FUNCTION_BLOCK PQDXXA_PARA
TITLE =PN Driver
AUTHOR : Parker
VERSION : 0.2


VAR_INPUT
  INIT : BOOL ;	//initilaize after Start / Baustein initialisieren
  READ_ALL : BOOL ;	//read out all parameters / alle Parameter auslesen
  WRITE_ALL : BOOL ;	//write all parameters / alle Parameter schreiben
  WRITE_SEL : BOOL ;	//write only selection parameters / nur die Auswahlparameter schreiben
  SINGLE_READ : BOOL ;	//read single parameter / einzelnen Wert lesen
  SINGLE_WRITE : BOOL ;	//write single parameter / einezelnen Wert schreiben
  SINGLE_INDEX : WORD ;	//parameter address / Adresse
  SAVE : BOOL ;	//save parameters in the module / Parameter im Modul speichern
  DEFAULT : BOOL ;	//set all parameters to the default setting / alle Parameter auf Werkseinstellung
  LOADBACK : BOOL ;	//load back the last saved parameter set / letzten gespeicheten Parametersatz zur
  PAR_CHANGE_OUT : STRUCT
   PARA_READY : BOOL ;
   BUS_VALID : BOOL ;
   ENABLE : BOOL ;	//Enable Signal for the Controller
   PARA_ACTIVE : BOOL ;
   PARVAL : DWORD ;	//Read out Value
  END_STRUCT ;
END_VAR
VAR_OUTPUT
  STATUS : INT ;	//0 = no active, 1 = ready and intitialized, 2 = busy, 3 = error / 0 = inaktiv, 1
  ERROR_LINE : INT ;	//number of the faulty parameter (range test or timeout) / Nummer des fehlerhafte
  DISC_LINE : INT ;	//line of 1st deviation / Zeile mit der ersten Abweichung
  DISC_COUNT : INT ;	//number of deriving parameters / Zahl der abweichenden Parameter
  PAR_CHANGE_IN : STRUCT
   PARVAL : DWORD ;
   PARAMODE : BOOL ;
   ADDRESS : WORD ;
   PARAVALID : BOOL ;
   PARAREAD : BOOL ;
   READULIM : BOOL ;
   READLLIM : BOOL ;
  END_STRUCT ;
END_VAR
VAR_IN_OUT
  PVSEL : INT ;	//Pump displacement selection [cm³/rev] / Auswahl des Verdrängungsvolumen [cm³/re
  PTYPE : INT ;	//1=F (swivel angle ctrl.), 2=P (+ open loop pressure ctrl.), 3=Q (+ closed loop
  CO : INT ;	//Selection of control option: 1=FP*/UP*, 2=FD*/UD* / Auswahl der Regleroption: 1
  DSP_VALVE : INT ;	//Pressure valve design series 2 = "11", 1 = "12"/ Konstruktionsstand des Druckve
  PSENSOR : INT ;	//Sensor nominal pressure in bar / Sensor Nenndruck in bar
  PNOMINAL : INT ;	//System pressure value in bar / Systemdruck in bar
  PCORR : INT ;	//Differential pressure setting in bar / Differenzdruckeinstellung in bar
  PLRPM : INT ;	//Engine speed in rpm / Motordrehzahl in U/min
  PLPL : INT ;	//Power limitation in 0,1kW / Leistungsgrenze in 0,1kW
  QCORR : INT ;	//Automatic flow correction in 0,01% / Automatische Volumenstromkorrektur in 0,01
  AQUP : DINT ;	//Ramp time up stroking (flow) for 0... 100% in ms / Rampenzeit aufschwenken (Vol
  AQDOWN : DINT ;	//Ramp time down stroking (flow) for 0... 100% in ms / Rampenzeit abschwenken (Vo
  APUP : DINT ;	//Ramp time (pressure up) for 0... 100% in ms / Rampenzeit (Druckanstieg) für 0..
  APDOWN : DINT ;	//Ramp time (pressure down) for 0... 100% in ms / Rampenzeit (Druckreduzierung) f
  MINXQ : INT ;	//Input scaling of the swivel angle sensor signal in mV / Eingangsskalierung des
  MAXXQ : INT ;	//Input scaling of the swivel angle sensor signal in mV / Eingangsskalierung des
  AINXQ : INT ;	//Input signal switching, swivel angel sensor, voltage (1) or current (2)/ Eingan
  AINXP : INT ;	//Input signal switching pressure sensor, voltage (1) or current (2) / Eingangssi
  CQFF : INT ;	//Offset swivel angle controller in 0,01% / Offset des Schwenkwinkelreglers in 0,
  CQP : INT ;	//P gain in 0,01 units / P-Anteil, Verstärkung in 0,01 Einheiten
  CQI : INT ;	//I gain in 0,1ms / I-Anteil, Nachstellzeit in 0,1ms
  CQILIM : INT ;	//I gain limitation in 0,01% / I-Anteil, Begegrenzung in 0,01%
  CQIC : INT ;	//I gain activation in 0,01% / I-Anteil, Aktivierung in 0,01%
  CQD : INT ;	//D gain in 0,1ms / D-Anteil, Vorhaltezeit in 0,1ms
  CQT1 : INT ;	//D gain filter in 0,1ms / D-Anteil, Filter in 0,1ms
  CPFF : INT ;	//Feed forward pressure valve in 0,01% / Vorsteuerwert des Druckventils in 0,01%
  CPP : INT ;	//P gain in 0,01 units / P-Anteil, Verstärkung in 0,01 Einheiten
  CPI : INT ;	//I gain in 0,1ms / I-Anteil, Nachstellzeit in 0,1ms
  CPILIM : INT ;	//I gain limitation in 0,01% / I-Anteil, Begrenzung in 0,01%
  CPIC : INT ;	//I gain activation in 0,01% / I-Anteil, Aktivierung in 0,01%
  CPD : INT ;	//D gain in 0,1ms / D-Anteil, Vorhaltezeit in 0,1ms
  CPT1 : INT ;	//D gain filter in 0,1ms / D-Anteil, Filter in 0,1ms
  CQMINVA : INT ;	//Compensation of the swivel angle valve deadband in mA / Kompensation der positi
  CQMINVB : INT ;	//Compensation of the swivel angle valve deadband in mA / Kompensation der positi
  CQMAXVA : INT ;	//Nominal current of the swivel angle valve in mA / Nennstrom des Schwenkwinkelve
  CQMAXVB : INT ;	//Nominal current of the swivel angle valve in mA / Nennstrom des Schwenkwinkelve
  TRIGGERQ : INT ;	//Trigger point of the swivel angel valve MIN function in 0,01% / Triggerpunkt de
  OFFSETQ : INT ;	//Offset function for neutral point adjustment of the directional valve in 0,01%
  CPMINV : INT ;	//Response threshold of the pressure valve in mA / Ansprechschwelle des Druckvent
  CPMAXV : INT ;	//Nominal current of the pressure valve in mA / Nennstrom des Druckventils in mA
  TRIGGERP : INT ;	//Trigger point of the pressure valve MIN function in 0,01% / Triggerpunkt der MI
  DFREQQ : INT ;	//Dither frequency in Hz / Dither Frequenz in Hz
  DAMPLQ : INT ;	//Dither amplitude in 0,01% of the rated current / Dither Amplitude in 0,01% des
  PWMQ : INT ;	//PWM Frequenz in Hz: 1-17 = 100|120|150|200|269|372|488|624|781|976|1201|1420|15
  PPWMQ : INT ;	//P gain of the current controller / P Verstärkung des Stromreglers
  IPWMQ : INT ;	//I gain of the current controller / I Verstärkung des Stromreglers
  DFREQP : INT ;	//Dither frequency in Hz / Dither Frequenz in Hz
  DAMPLP : INT ;	//Dither amplitude in 0,01% of the rated current / Dither Amplitude in 0,01% des
  PWMP : INT ;	//PWM Frequenz in Hz: 1-17 = 100|120|150|200|269|372|488|624|781|976|1201|1420|15
  PPWMP : INT ;	//P gain of the current controller / P Verstärkung des Stromreglers
  IPWMP : INT ;	//I gain of the current controller / I Verstärkung des Stromreglers
  SINGLEACCESS : DINT ;
END_VAR
VAR
  PARAINFO : ARRAY  [1 .. 51 ] OF STRUCT
   MINV : INT ;
   MAXV : INT ;
   VALUE : INT ;
   ADDRESS : WORD  := W#16#2001;
  END_STRUCT ;
  PARAINFO_LONG : ARRAY  [1 .. 4 ] OF STRUCT
   MINV : DINT ;
   MAXV : DINT ;
   VALUE : DINT ;
  END_STRUCT ;
  INTERNAL_STATE : INT ;
  SUBSTATE : INT ;
  i : INT ;
  actWaitCycles : INT ;
  oldParaReadVal : DWORD ;
  oldREADALL : BOOL ;
  oldWRITESEL : BOOL ;
  oldWRITEALL : BOOL ;
  oldPARAREADY : BOOL ;
  oldSINGLEWRITE : BOOL ;
  oldSINGLEREAD : BOOL ;
  oldSAVE : BOOL ;
  oldDEFAULT : BOOL ;
  oldLOADBACK : BOOL ;
  defaultFlag : BOOL ;
  saveFlag : BOOL ;
  readInEAFlag : BOOL ;
  readOnlyValues : BOOL ;
  initReceived : BOOL ;
  writeLimit : INT ;
  copyValue : INT ;
  copyValueLong : DINT ;
  discCountTemp : INT ;
  Displacement : ARRAY  [1 .. 15 ] OF
  INT  := 16, 20, 23, 28, 32, 40, 46, 63, 80, 92, 140, 180, 270, 360, 0;
END_VAR
VAR_TEMP
  MemFkt : INT ;
  PCI_DEFAULT : STRUCT
   PARVAL : DWORD ;
   PARAMODE : BOOL ;
   ADDRESS : WORD ;
   PARAVALID : BOOL ;
   PARAREAD : BOOL ;
   READULIM : BOOL ;
   READLLIM : BOOL ;
  END_STRUCT ;
  k : INT ;
  tmpDiff : DINT ;
  repeatFlag : BOOL ;
  tmpBool : BOOL ;
END_VAR
BEGIN
NETWORK
TITLE =SCL network
      SET   ;
      SAVE  ;
      =     L     18.3;
A7d0: CLR   ;
      =     #repeatFlag;
      U     #PAR_CHANGE_OUT.BUS_VALID;
      NOT   ;
      SPBN  A7d1;
      L     5;
      T     #INTERNAL_STATE;
      L     0;
      T     #SUBSTATE;
A7d1: L     #INTERNAL_STATE;
      L     20;
      <>I   ;
      SPBN  A7d2;
      L     0;
      T     #DISC_COUNT;
      L     -1;
      T     #DISC_LINE;
A7d2: CLR   ;
      U     #initReceived;
      NOT   ;
      U     #INIT;
      SPBN  A7d3;
      L     0;
      T     #INTERNAL_STATE;
      SET   ;
      =     #initReceived;
A7d3: L     #INTERNAL_STATE;
      L     0;
      TAK   ;
      ==I   ;
      T     LW    20;
      SPB   A7d5;
      SPA   A7d6;
A7d5: L     W#16#2001;
      T     #PARAINFO[1].ADDRESS;
      L     W#16#2002;
      T     #PARAINFO[2].ADDRESS;
      L     W#16#2003;
      T     #PARAINFO[3].ADDRESS;
      L     W#16#2004;
      T     #PARAINFO[4].ADDRESS;
      L     W#16#2011;
      T     #PARAINFO[5].ADDRESS;
      L     W#16#2012;
      T     #PARAINFO[6].ADDRESS;
      L     W#16#2013;
      T     #PARAINFO[7].ADDRESS;
      L     W#16#2014;
      T     #PARAINFO[8].ADDRESS;
      L     W#16#2015;
      T     #PARAINFO[9].ADDRESS;
      L     W#16#2016;
      T     #PARAINFO[10].ADDRESS;
      L     W#16#2021;
      T     #PARAINFO[11].ADDRESS;
      L     W#16#2022;
      T     #PARAINFO[12].ADDRESS;
      L     W#16#2023;
      T     #PARAINFO[13].ADDRESS;
      L     W#16#2024;
      T     #PARAINFO[14].ADDRESS;
      L     W#16#2025;
      T     #PARAINFO[15].ADDRESS;
      L     W#16#2026;
      T     #PARAINFO[16].ADDRESS;
      L     W#16#2027;
      T     #PARAINFO[17].ADDRESS;
      L     W#16#2028;
      T     #PARAINFO[18].ADDRESS;
      L     W#16#2031;
      T     #PARAINFO[19].ADDRESS;
      L     W#16#2032;
      T     #PARAINFO[20].ADDRESS;
      L     W#16#2033;
      T     #PARAINFO[21].ADDRESS;
      L     W#16#2034;
      T     #PARAINFO[22].ADDRESS;
      L     W#16#2039;
      T     #PARAINFO[23].ADDRESS;
      L     W#16#2036;
      T     #PARAINFO[24].ADDRESS;
      L     W#16#2037;
      T     #PARAINFO[25].ADDRESS;
      L     W#16#2041;
      T     #PARAINFO[26].ADDRESS;
      L     W#16#2042;
      T     #PARAINFO[27].ADDRESS;
      L     W#16#2043;
      T     #PARAINFO[28].ADDRESS;
      L     W#16#2044;
      T     #PARAINFO[29].ADDRESS;
      L     W#16#2045;
      T     #PARAINFO[30].ADDRESS;
      L     W#16#2046;
      T     #PARAINFO[31].ADDRESS;
      L     W#16#2047;
      T     #PARAINFO[32].ADDRESS;
      L     W#16#2051;
      T     #PARAINFO[33].ADDRESS;
      L     W#16#2052;
      T     #PARAINFO[34].ADDRESS;
      L     W#16#2053;
      T     #PARAINFO[35].ADDRESS;
      L     W#16#2054;
      T     #PARAINFO[36].ADDRESS;
      L     W#16#2055;
      T     #PARAINFO[37].ADDRESS;
      L     W#16#2056;
      T     #PARAINFO[38].ADDRESS;
      L     W#16#2061;
      T     #PARAINFO[39].ADDRESS;
      L     W#16#2062;
      T     #PARAINFO[40].ADDRESS;
      L     W#16#2063;
      T     #PARAINFO[41].ADDRESS;
      L     W#16#2071;
      T     #PARAINFO[42].ADDRESS;
      L     W#16#2072;
      T     #PARAINFO[43].ADDRESS;
      L     W#16#2073;
      T     #PARAINFO[44].ADDRESS;
      L     W#16#2074;
      T     #PARAINFO[45].ADDRESS;
      L     W#16#2075;
      T     #PARAINFO[46].ADDRESS;
      L     W#16#2081;
      T     #PARAINFO[47].ADDRESS;
      L     W#16#2082;
      T     #PARAINFO[48].ADDRESS;
      L     W#16#2083;
      T     #PARAINFO[49].ADDRESS;
      L     W#16#2084;
      T     #PARAINFO[50].ADDRESS;
      L     W#16#2085;
      T     #PARAINFO[51].ADDRESS;
      CLR   ;
      =     #saveFlag;
      L     5;
      T     #INTERNAL_STATE;
      SPA   A7d4;
A7d6: L     5;
      L     LW    20;
      ==I   ;
      SPB   A7d7;
      SPA   A7d8;
A7d7: CLR   ;
      U     #PAR_CHANGE_OUT.BUS_VALID;
      SPBN  A7d9;
      L     8;
      T     #INTERNAL_STATE;
      L     0;
      T     #actWaitCycles;
      CLR   ;
      =     #readOnlyValues;
      T     #SUBSTATE;
      L     1;
      T     #i;
A7d9: L     0;
      T     #STATUS;
      L     #PCI_DEFAULT.PARVAL;
      T     #PAR_CHANGE_IN.PARVAL;
      L     LD     6;
      T     DID [AR2,P#24.0];
      L     LW    10;
      T     DIW [AR2,P#28.0];
      CLR   ;
      =     #readInEAFlag;
      SPA   A7d4;
A7d8: L     8;
      L     LW    20;
      ==I   ;
      SPB   A7da;
      SPA   A7db;
A7da: L     #actWaitCycles;
      L     100;
      <I    ;
      SPBN  A7dc;
      L     #actWaitCycles;
      L     1;
      +I    ;
      SPO   I007;
      SPA   I008;
I007: CLR   ;
      =     L     18.3;
I008: T     #actWaitCycles;
      SPA   A7d4;
A7dc: L     0;
      T     #actWaitCycles;
      L     10;
      T     #INTERNAL_STATE;
      SPA   A7d4;
A7db: L     10;
      L     LW    20;
      ==I   ;
      SPB   A7de;
      SPA   A7df;
A7de: L     2;
      T     #STATUS;
      L     #SUBSTATE;
      L     0;
      TAK   ;
      ==I   ;
      T     LW    22;
      SPB   A7e1;
      SPA   A7e2;
A7e1: L     #i;
      ITD   ;
      L     L#1;
      >=D   ;
      U     L     18.3;
      =     L     18.3;
      TAK   ;
      L     L#51;
      <=D   ;
      U     L     18.3;
      =     L     18.3;
      TAK   ;
      L     L#1;
      -D    ;
      SPO   I009;
      SPA   I00a;
I009: CLR   ;
      =     L     18.3;
I00a: L     L#64;
      *D    ;
      SPO   I00b;
      SPA   I00c;
I00b: CLR   ;
      =     L     18.3;
I00c: L     L#48;
      +D    ;
      SPO   I00d;
      SPA   I00e;
I00d: CLR   ;
      =     L     18.3;
I00e: TAR2  ;
      +D    ;
      SPO   I00f;
      SPA   I010;
I00f: CLR   ;
      =     L     18.3;
I010: LAR1  ;
      L     DIW [AR1,P#144.0];
      T     #PAR_CHANGE_IN.ADDRESS;
      CLR   ;
      U     #readOnlyValues;
      SPBN  A7e3;
      L     40;
      T     #SUBSTATE;
      SPA   A7e0;
A7e3: SET   ;
      =     #PAR_CHANGE_IN.READLLIM;
      =     #PAR_CHANGE_IN.PARAREAD;
      L     0;
      T     #actWaitCycles;
      L     #PAR_CHANGE_OUT.PARVAL;
      T     #oldParaReadVal;
      L     10;
      T     #SUBSTATE;
      SPA   A7e0;
A7e2: L     10;
      L     LW    22;
      ==I   ;
      SPB   A7e5;
      SPA   A7e6;
A7e5: L     #PAR_CHANGE_OUT.PARVAL;
      L     #oldParaReadVal;
      <>D   ;
      L     #actWaitCycles;
      L     5;
      =     L     18.4;
      >=I   ;
      O     L     18.4;
      SPBN  A7e7;
      L     #i;
      L     11;
      <I    ;
      L     #i;
      L     14;
      =     L     18.4;
      >I    ;
      O     L     18.4;
      SPBN  A7e8;
      L     #i;
      ITD   ;
      L     L#1;
      >=D   ;
      U     L     18.3;
      =     L     18.3;
      TAK   ;
      L     L#51;
      <=D   ;
      U     L     18.3;
      =     L     18.3;
      TAK   ;
      L     L#1;
      -D    ;
      SPO   I011;
      SPA   I012;
I011: CLR   ;
      =     L     18.3;
I012: L     L#64;
      *D    ;
      SPO   I013;
      SPA   I014;
I013: CLR   ;
      =     L     18.3;
I014: TAR2  ;
      +D    ;
      SPO   I015;
      SPA   I016;
I015: CLR   ;
      =     L     18.3;
I016: L     #PAR_CHANGE_OUT.PARVAL;
      TAK   ;
      T     LD    24;
      TAK   ;
      PUSH  ;
      UD    DW#16#FFFF0000;
      TAK   ;
      SPZ   I017;
      CLR   ;
      =     L     18.3;
I017: CLR   ;
      U     L     18.3;
      SAVE  ;
      LAR1  LD    24;
      T     DIW [AR1,P#144.0];
      SPA   A7e9;
A7e8: L     #i;
      L     -10;
      +I    ;
      SPO   I018;
      SPA   I019;
I018: CLR   ;
      =     L     18.3;
I019: ITD   ;
      L     L#1;
      >=D   ;
      U     L     18.3;
      =     L     18.3;
      TAK   ;
      L     L#4;
      <=D   ;
      U     L     18.3;
      =     L     18.3;
      TAK   ;
      L     L#1;
      -D    ;
      SPO   I01a;
      SPA   I01b;
I01a: CLR   ;
      =     L     18.3;
I01b: L     L#96;
      *D    ;
      SPO   I01c;
      SPA   I01d;
I01c: CLR   ;
      =     L     18.3;
I01d: TAR2  ;
      +D    ;
      SPO   I01e;
      SPA   I01f;
I01e: CLR   ;
      =     L     18.3;
I01f: L     #PAR_CHANGE_OUT.PARVAL;
      CLR   ;
      U     L     18.3;
      SAVE  ;
      TAK   ;
      LAR1  ;
      TAK   ;
      T     DID [AR1,P#552.0];
A7e9: L     20;
      T     #SUBSTATE;
      CLR   ;
      =     #PAR_CHANGE_IN.PARAREAD;
      L     0;
      T     #actWaitCycles;
      SPA   A7e0;
A7e7: L     #actWaitCycles;
      L     1;
      +I    ;
      SPO   I020;
      SPA   I021;
I020: CLR   ;
      =     L     18.3;
I021: T     #actWaitCycles;
      SPA   A7e0;
A7e6: L     20;
      L     LW    22;
      ==I   ;
      SPB   A7eb;
      SPA   A7ec;
A7eb: L     #actWaitCycles;
      L     5;
      >=I   ;
      SPBN  A7ed;
      CLR   ;
      =     #PAR_CHANGE_IN.READLLIM;
      SET   ;
      =     #PAR_CHANGE_IN.READULIM;
      =     #PAR_CHANGE_IN.PARAREAD;
      L     0;
      T     #actWaitCycles;
      L     #PAR_CHANGE_OUT.PARVAL;
      T     #oldParaReadVal;
      L     30;
      T     #SUBSTATE;
      SPA   A7e0;
A7ed: L     #actWaitCycles;
      L     1;
      +I    ;
      SPO   I022;
      SPA   I023;
I022: CLR   ;
      =     L     18.3;
I023: T     #actWaitCycles;
      SPA   A7e0;
A7ec: L     30;
      L     LW    22;
      ==I   ;
      SPB   A7ef;
      SPA   A7f0;
A7ef: L     #PAR_CHANGE_OUT.PARVAL;
      L     #oldParaReadVal;
      <>D   ;
      L     #actWaitCycles;
      L     5;
      =     L     18.4;
      >=I   ;
      O     L     18.4;
      SPBN  A7f1;
      L     #i;
      L     11;
      <I    ;
      L     #i;
      L     14;
      =     L     18.4;
      >I    ;
      O     L     18.4;
      SPBN  A7f2;
      L     #i;
      ITD   ;
      L     L#1;
      >=D   ;
      U     L     18.3;
      =     L     18.3;
      TAK   ;
      L     L#51;
      <=D   ;
      U     L     18.3;
      =     L     18.3;
      TAK   ;
      L     L#1;
      -D    ;
      SPO   I024;
      SPA   I025;
I024: CLR   ;
      =     L     18.3;
I025: L     L#64;
      *D    ;
      SPO   I026;
      SPA   I027;
I026: CLR   ;
      =     L     18.3;
I027: L     L#16;
      +D    ;
      SPO   I028;
      SPA   I029;
I028: CLR   ;
      =     L     18.3;
I029: TAR2  ;
      +D    ;
      SPO   I02a;
      SPA   I02b;
I02a: CLR   ;
      =     L     18.3;
I02b: L     #PAR_CHANGE_OUT.PARVAL;
      TAK   ;
      T     LD    24;
      TAK   ;
      PUSH  ;
      UD    DW#16#FFFF0000;
      TAK   ;
      SPZ   I02c;
      CLR   ;
      =     L     18.3;
I02c: CLR   ;
      U     L     18.3;
      SAVE  ;
      LAR1  LD    24;
      T     DIW [AR1,P#144.0];
      SPA   A7f3;
A7f2: L     #i;
      L     -10;
      +I    ;
      SPO   I02d;
      SPA   I02e;
I02d: CLR   ;
      =     L     18.3;
I02e: ITD   ;
      L     L#1;
      >=D   ;
      U     L     18.3;
      =     L     18.3;
      TAK   ;
      L     L#4;
      <=D   ;
      U     L     18.3;
      =     L     18.3;
      TAK   ;
      L     L#1;
      -D    ;
      SPO   I02f;
      SPA   I030;
I02f: CLR   ;
      =     L     18.3;
I030: L     L#96;
      *D    ;
      SPO   I031;
      SPA   I032;
I031: CLR   ;
      =     L     18.3;
I032: L     L#32;
      +D    ;
      SPO   I033;
      SPA   I034;
I033: CLR   ;
      =     L     18.3;
I034: TAR2  ;
      +D    ;
      SPO   I035;
      SPA   I036;
I035: CLR   ;
      =     L     18.3;
I036: L     #PAR_CHANGE_OUT.PARVAL;
      CLR   ;
      U     L     18.3;
      SAVE  ;
      TAK   ;
      LAR1  ;
      TAK   ;
      T     DID [AR1,P#552.0];
A7f3: L     40;
      T     #SUBSTATE;
      CLR   ;
      =     #PAR_CHANGE_IN.PARAREAD;
      L     0;
      T     #actWaitCycles;
      SPA   A7e0;
A7f1: L     #actWaitCycles;
      L     1;
      +I    ;
      SPO   I037;
      SPA   I038;
I037: CLR   ;
      =     L     18.3;
I038: T     #actWaitCycles;
      SPA   A7e0;
A7f0: L     40;
      L     LW    22;
      ==I   ;
      SPB   A7f5;
      SPA   A7f6;
A7f5: L     #actWaitCycles;
      L     5;
      >=I   ;
      SPBN  A7f7;
      CLR   ;
      =     #PAR_CHANGE_IN.READLLIM;
      =     #PAR_CHANGE_IN.READULIM;
      SET   ;
      =     #PAR_CHANGE_IN.PARAREAD;
      L     0;
      T     #actWaitCycles;
      L     #PAR_CHANGE_OUT.PARVAL;
      T     #oldParaReadVal;
      L     50;
      T     #SUBSTATE;
      SPA   A7e0;
A7f7: L     #actWaitCycles;
      L     1;
      +I    ;
      SPO   I039;
      SPA   I03a;
I039: CLR   ;
      =     L     18.3;
I03a: T     #actWaitCycles;
      SPA   A7e0;
A7f6: L     50;
      L     LW    22;
      ==I   ;
      SPB   A7f9;
      SPA   A7fa;
A7f9: L     #PAR_CHANGE_OUT.PARVAL;
      L     #oldParaReadVal;
      <>D   ;
      L     #actWaitCycles;
      L     5;
      =     L     18.4;
      >=I   ;
      O     L     18.4;
      SPBN  A7fb;
      L     #i;
      L     11;
      <I    ;
      L     #i;
      L     14;
      =     L     18.4;
      >I    ;
      O     L     18.4;
      SPBN  A7fc;
      L     #i;
      ITD   ;
      L     L#1;
      >=D   ;
      U     L     18.3;
      =     L     18.3;
      TAK   ;
      L     L#51;
      <=D   ;
      U     L     18.3;
      =     L     18.3;
      TAK   ;
      L     L#1;
      -D    ;
      SPO   I03b;
      SPA   I03c;
I03b: CLR   ;
      =     L     18.3;
I03c: L     L#64;
      *D    ;
      SPO   I03d;
      SPA   I03e;
I03d: CLR   ;
      =     L     18.3;
I03e: L     L#32;
      +D    ;
      SPO   I03f;
      SPA   I040;
I03f: CLR   ;
      =     L     18.3;
I040: TAR2  ;
      +D    ;
      SPO   I041;
      SPA   I042;
I041: CLR   ;
      =     L     18.3;
I042: L     #PAR_CHANGE_OUT.PARVAL;
      TAK   ;
      T     LD    24;
      TAK   ;
      PUSH  ;
      UD    DW#16#FFFF0000;
      TAK   ;
      SPZ   I043;
      CLR   ;
      =     L     18.3;
I043: CLR   ;
      U     L     18.3;
      SAVE  ;
      LAR1  LD    24;
      T     DIW [AR1,P#144.0];
      SPA   A7fd;
A7fc: L     #i;
      L     -10;
      +I    ;
      SPO   I044;
      SPA   I045;
I044: CLR   ;
      =     L     18.3;
I045: ITD   ;
      L     L#1;
      >=D   ;
      U     L     18.3;
      =     L     18.3;
      TAK   ;
      L     L#4;
      <=D   ;
      U     L     18.3;
      =     L     18.3;
      TAK   ;
      L     L#1;
      -D    ;
      SPO   I046;
      SPA   I047;
I046: CLR   ;
      =     L     18.3;
I047: L     L#96;
      *D    ;
      SPO   I048;
      SPA   I049;
I048: CLR   ;
      =     L     18.3;
I049: L     L#64;
      +D    ;
      SPO   I04a;
      SPA   I04b;
I04a: CLR   ;
      =     L     18.3;
I04b: TAR2  ;
      +D    ;
      SPO   I04c;
      SPA   I04d;
I04c: CLR   ;
      =     L     18.3;
I04d: L     #PAR_CHANGE_OUT.PARVAL;
      CLR   ;
      U     L     18.3;
      SAVE  ;
      TAK   ;
      LAR1  ;
      TAK   ;
      T     DID [AR1,P#552.0];
A7fd: CLR   ;
      =     #PAR_CHANGE_IN.PARAREAD;
      L     0;
      T     #actWaitCycles;
      L     55;
      T     #SUBSTATE;
      U     #readInEAFlag;
      SPBN  A7e0;
      L     2;
      T     #MemFkt;
      L     #i;
      L     11;
      <I    ;
      L     #i;
      L     14;
      =     L     18.4;
      >I    ;
      O     L     18.4;
      SPBN  A7ff;
      L     #i;
      ITD   ;
      L     L#1;
      >=D   ;
      U     L     18.3;
      =     L     18.3;
      TAK   ;
      L     L#51;
      <=D   ;
      U     L     18.3;
      =     L     18.3;
      TAK   ;
      L     L#1;
      -D    ;
      SPO   I04e;
      SPA   I04f;
I04e: CLR   ;
      =     L     18.3;
I04f: L     L#64;
      *D    ;
      SPO   I050;
      SPA   I051;
I050: CLR   ;
      =     L     18.3;
I051: L     L#32;
      +D    ;
      SPO   I052;
      SPA   I053;
I052: CLR   ;
      =     L     18.3;
I053: TAR2  ;
      +D    ;
      SPO   I054;
      SPA   I055;
I054: CLR   ;
      =     L     18.3;
I055: LAR1  ;
      L     DIW [AR1,P#144.0];
      T     #copyValue;
      SPA   A800;
A7ff: L     #PAR_CHANGE_OUT.PARVAL;
      T     #copyValueLong;
      CLR   ;
      U     L     18.3;
      SAVE  ;
A800: SPA   A7e0;
A7fb: L     #actWaitCycles;
      L     1;
      +I    ;
      SPO   I056;
      SPA   I057;
I056: CLR   ;
      =     L     18.3;
I057: T     #actWaitCycles;
      SPA   A7e0;
A7fa: L     55;
      L     LW    22;
      ==I   ;
      SPB   A802;
      SPA   A7e0;
A802: L     #i;
      L     51;
      >=I   ;
      SPBN  A804;
      L     20;
      T     #INTERNAL_STATE;
      L     1;
      T     #i;
      L     #PCI_DEFAULT.PARVAL;
      T     #PAR_CHANGE_IN.PARVAL;
      L     LD     6;
      T     DID [AR2,P#24.0];
      L     LW    10;
      T     DIW [AR2,P#28.0];
      CLR   ;
      =     #readInEAFlag;
      L     1;
      T     #STATUS;
      SPA   A805;
A804: L     #i;
      L     1;
      +I    ;
      SPO   I058;
      SPA   I059;
I058: CLR   ;
      =     L     18.3;
I059: T     #i;
A805: L     0;
      T     #SUBSTATE;
A7e0: SPA   A7d4;
A7df: L     20;
      L     LW    20;
      ==I   ;
      SPB   A806;
      SPA   A807;
A806: CLR   ;
      U     #oldREADALL;
      NOT   ;
      U     #READ_ALL;
      SPBN  A808;
      L     10;
      T     #INTERNAL_STATE;
      CLR   ;
      =     #readOnlyValues;
      SET   ;
      =     #readInEAFlag;
      L     0;
      T     #ERROR_LINE;
      L     1;
      T     #i;
      SPA   A809;
A808: CLR   ;
      U     #oldWRITESEL;
      NOT   ;
      U     #WRITE_SEL;
      SPBN  A80a;
      U     #PAR_CHANGE_OUT.ENABLE;
      SPBN  A80b;
      L     3;
      T     #STATUS;
      SPA   A809;
A80b: L     30;
      T     #INTERNAL_STATE;
      L     0;
      T     #ERROR_LINE;
      L     4;
      T     #writeLimit;
      SET   ;
      =     #readInEAFlag;
      L     1;
      T     #i;
      SPA   A809;
A80a: CLR   ;
      U     #oldWRITEALL;
      NOT   ;
      U     #WRITE_ALL;
      SPBN  A80d;
      U     #PAR_CHANGE_OUT.ENABLE;
      SPBN  A80e;
      L     3;
      T     #STATUS;
      SPA   A809;
A80e: L     30;
      T     #INTERNAL_STATE;
      L     0;
      T     #ERROR_LINE;
      L     51;
      T     #writeLimit;
      L     1;
      T     #i;
      SPA   A809;
A80d: CLR   ;
      U     #oldSINGLEREAD;
      NOT   ;
      U     #SINGLE_READ;
      SPBN  A810;
      L     40;
      T     #INTERNAL_STATE;
      L     0;
      T     #ERROR_LINE;
      SPA   A809;
A810: CLR   ;
      U     #oldSINGLEWRITE;
      NOT   ;
      U     #SINGLE_WRITE;
      SPBN  A811;
      L     50;
      T     #INTERNAL_STATE;
      L     0;
      T     #ERROR_LINE;
      SPA   A809;
A811: CLR   ;
      U     #oldSAVE;
      NOT   ;
      U     #SAVE;
      SPBN  A812;
      L     50;
      T     #INTERNAL_STATE;
      SET   ;
      =     #saveFlag;
      L     0;
      T     #ERROR_LINE;
      SPA   A809;
A812: CLR   ;
      U     #oldDEFAULT;
      NOT   ;
      U     #DEFAULT;
      SPBN  A813;
      U     #PAR_CHANGE_OUT.ENABLE;
      SPBN  A814;
      L     3;
      T     #STATUS;
      SPA   A809;
A814: L     60;
      T     #INTERNAL_STATE;
      SET   ;
      =     #defaultFlag;
      =     #readInEAFlag;
      L     0;
      T     #ERROR_LINE;
      SPA   A809;
A813: CLR   ;
      U     #oldLOADBACK;
      NOT   ;
      U     #LOADBACK;
      SPBN  A816;
      U     #PAR_CHANGE_OUT.ENABLE;
      SPBN  A817;
      L     3;
      T     #STATUS;
      SPA   A809;
A817: L     60;
      T     #INTERNAL_STATE;
      CLR   ;
      =     #defaultFlag;
      SET   ;
      =     #readInEAFlag;
      L     0;
      T     #ERROR_LINE;
      SPA   A809;
A816: L     #i;
      L     11;
      <I    ;
      L     #i;
      L     14;
      =     L     18.4;
      >I    ;
      O     L     18.4;
      SPBN  A819;
      L     #i;
      ITD   ;
      L     L#1;
      >=D   ;
      U     L     18.3;
      =     L     18.3;
      TAK   ;
      L     L#51;
      <=D   ;
      U     L     18.3;
      =     L     18.3;
      TAK   ;
      L     L#1;
      -D    ;
      SPO   I05a;
      SPA   I05b;
I05a: CLR   ;
      =     L     18.3;
I05b: L     L#64;
      *D    ;
      SPO   I05c;
      SPA   I05d;
I05c: CLR   ;
      =     L     18.3;
I05d: L     L#32;
      +D    ;
      SPO   I05e;
      SPA   I05f;
I05e: CLR   ;
      =     L     18.3;
I05f: TAR2  ;
      +D    ;
      SPO   I060;
      SPA   I061;
I060: CLR   ;
      =     L     18.3;
I061: L     #copyValue;
      TAK   ;
      LAR1  ;
      TAK   ;
      L     DIW [AR1,P#144.0];
      -I    ;
      SPO   I062;
      SPA   I063;
I062: CLR   ;
      =     L     18.3;
I063: L     W#16#0;
      >=I   ;
      TAK   ;
      SPB   I064;
      NEGI  ;
      SPO   I065;
      SPA   I064;
I065: CLR   ;
      =     L     18.3;
I064: CLR   ;
      U     L     18.3;
      SAVE  ;
      ITD   ;
      T     #tmpDiff;
      L     #i;
      ITD   ;
      L     L#1;
      >=D   ;
      U     L     18.3;
      =     L     18.3;
      TAK   ;
      L     L#51;
      <=D   ;
      U     L     18.3;
      =     L     18.3;
      TAK   ;
      L     L#1;
      -D    ;
      SPO   I066;
      SPA   I067;
I066: CLR   ;
      =     L     18.3;
I067: L     L#64;
      *D    ;
      SPO   I068;
      SPA   I069;
I068: CLR   ;
      =     L     18.3;
I069: L     L#16;
      +D    ;
      SPO   I06a;
      SPA   I06b;
I06a: CLR   ;
      =     L     18.3;
I06b: TAR2  ;
      +D    ;
      SPO   I06c;
      SPA   I06d;
I06c: CLR   ;
      =     L     18.3;
I06d: L     #i;
      ITD   ;
      TAK   ;
      T     LD    22;
      TAK   ;
      L     L#1;
      >=D   ;
      U     L     18.3;
      =     L     18.3;
      TAK   ;
      L     L#51;
      <=D   ;
      U     L     18.3;
      =     L     18.3;
      TAK   ;
      L     L#1;
      -D    ;
      SPO   I06e;
      SPA   I06f;
I06e: CLR   ;
      =     L     18.3;
I06f: L     L#64;
      *D    ;
      SPO   I070;
      SPA   I071;
I070: CLR   ;
      =     L     18.3;
I071: TAR2  ;
      +D    ;
      SPO   I072;
      SPA   I073;
I072: CLR   ;
      =     L     18.3;
I073: LAR1  LD    22;
      L     DIW [AR1,P#144.0];
      TAK   ;
      LAR1  ;
      TAK   ;
      L     DIW [AR1,P#144.0];
      -I    ;
      SPO   I074;
      SPA   I075;
I074: CLR   ;
      =     L     18.3;
I075: L     20;
      >I    ;
      SPBN  A81a;
      L     #tmpDiff;
      L     L#100;
      *D    ;
      SPO   I076;
      SPA   I077;
I076: CLR   ;
      =     L     18.3;
I077: L     #i;
      ITD   ;
      TAK   ;
      T     LD    22;
      TAK   ;
      L     L#1;
      >=D   ;
      U     L     18.3;
      =     L     18.3;
      TAK   ;
      L     L#51;
      <=D   ;
      U     L     18.3;
      =     L     18.3;
      TAK   ;
      L     L#1;
      -D    ;
      SPO   I078;
      SPA   I079;
I078: CLR   ;
      =     L     18.3;
I079: L     L#64;
      *D    ;
      SPO   I07a;
      SPA   I07b;
I07a: CLR   ;
      =     L     18.3;
I07b: L     L#32;
      +D    ;
      SPO   I07c;
      SPA   I07d;
I07c: CLR   ;
      =     L     18.3;
I07d: TAR2  ;
      +D    ;
      SPO   I07e;
      SPA   I07f;
I07e: CLR   ;
      =     L     18.3;
I07f: LAR1  ;
      L     DIW [AR1,P#144.0];
      T     LW    26;
      L     100;
      >=I   ;
      SPB   A81b;
      T     LW    26;
A81b: L     LW    26;
      ITD   ;
      L     LD    22;
      TAK   ;
      >D    ;
      =     #tmpBool;
      SPA   A81d;
A81a: L     #tmpDiff;
      L     L#0;
      <>D   ;
      =     #tmpBool;
      SPA   A81d;
A819: L     #i;
      L     -10;
      +I    ;
      SPO   I080;
      SPA   I081;
I080: CLR   ;
      =     L     18.3;
I081: ITD   ;
      L     L#1;
      >=D   ;
      U     L     18.3;
      =     L     18.3;
      TAK   ;
      L     L#4;
      <=D   ;
      U     L     18.3;
      =     L     18.3;
      TAK   ;
      L     L#1;
      -D    ;
      SPO   I082;
      SPA   I083;
I082: CLR   ;
      =     L     18.3;
I083: L     L#96;
      *D    ;
      SPO   I084;
      SPA   I085;
I084: CLR   ;
      =     L     18.3;
I085: L     L#64;
      +D    ;
      SPO   I086;
      SPA   I087;
I086: CLR   ;
      =     L     18.3;
I087: TAR2  ;
      +D    ;
      SPO   I088;
      SPA   I089;
I088: CLR   ;
      =     L     18.3;
I089: L     #copyValueLong;
      TAK   ;
      LAR1  ;
      TAK   ;
      L     DID [AR1,P#552.0];
      -D    ;
      SPO   I08a;
      SPA   I08b;
I08a: CLR   ;
      =     L     18.3;
I08b: L     DW#16#0;
      >=D   ;
      TAK   ;
      SPB   I08c;
      NEGD  ;
      SPO   I08d;
      SPA   I08c;
I08d: CLR   ;
      =     L     18.3;
I08c: T     #tmpDiff;
      CLR   ;
      U     L     18.3;
      SAVE  ;
      L     L#100;
      *D    ;
      SPO   I08e;
      SPA   I08f;
I08e: CLR   ;
      =     L     18.3;
I08f: L     #i;
      TAK   ;
      T     LD    22;
      TAK   ;
      L     -10;
      +I    ;
      SPO   I090;
      SPA   I091;
I090: CLR   ;
      =     L     18.3;
I091: ITD   ;
      L     L#1;
      >=D   ;
      U     L     18.3;
      =     L     18.3;
      TAK   ;
      L     L#4;
      <=D   ;
      U     L     18.3;
      =     L     18.3;
      TAK   ;
      L     L#1;
      -D    ;
      SPO   I092;
      SPA   I093;
I092: CLR   ;
      =     L     18.3;
I093: L     L#96;
      *D    ;
      SPO   I094;
      SPA   I095;
I094: CLR   ;
      =     L     18.3;
I095: L     L#64;
      +D    ;
      SPO   I096;
      SPA   I097;
I096: CLR   ;
      =     L     18.3;
I097: TAR2  ;
      +D    ;
      SPO   I098;
      SPA   I099;
I098: CLR   ;
      =     L     18.3;
I099: LAR1  ;
      L     DID [AR1,P#552.0];
      T     LD    26;
      L     L#100;
      >=D   ;
      SPB   A81e;
      T     LD    26;
A81e: L     LD    22;
      L     LD    26;
      >D    ;
      =     #tmpBool;
A81d: CLR   ;
      U     #tmpBool;
      SPBN  A81f;
      L     #discCountTemp;
      L     1;
      +I    ;
      SPO   I09a;
      SPA   I09b;
I09a: CLR   ;
      =     L     18.3;
I09b: T     #discCountTemp;
      L     1;
      ==I   ;
      SPBN  A81f;
      L     #i;
      T     #DISC_LINE;
A81f: L     #i;
      L     51;
      >=I   ;
      SPBN  A821;
      L     #discCountTemp;
      T     #DISC_COUNT;
      L     0;
      ==I   ;
      SPBN  A822;
      T     #DISC_LINE;
A822: L     1;
      T     #i;
      L     0;
      T     #discCountTemp;
      SPA   A823;
A821: L     #i;
      L     1;
      +I    ;
      SPO   I09c;
      SPA   I09d;
I09c: CLR   ;
      =     L     18.3;
I09d: T     #i;
A823: L     1;
      T     #MemFkt;
A809: L     #PCI_DEFAULT.PARVAL;
      T     #PAR_CHANGE_IN.PARVAL;
      L     LD     6;
      T     DID [AR2,P#24.0];
      L     LW    10;
      T     DIW [AR2,P#28.0];
      CLR   ;
      =     #initReceived;
      L     0;
      T     #SUBSTATE;
      SPA   A7d4;
A807: L     30;
      L     LW    20;
      ==I   ;
      SPB   A824;
      SPA   A825;
A824: L     #actWaitCycles;
      L     100;
      >=I   ;
      SPBN  A826;
      L     20;
      T     #INTERNAL_STATE;
      L     -1;
      T     #SUBSTATE;
      L     3;
      T     #STATUS;
      L     #i;
      T     #ERROR_LINE;
      CLR   ;
      =     #PAR_CHANGE_IN.PARAMODE;
      =     #PAR_CHANGE_IN.PARAVALID;
      SPA   A827;
A826: L     2;
      T     #STATUS;
A827: L     #SUBSTATE;
      L     0;
      TAK   ;
      ==I   ;
      T     LW    22;
      SPB   A829;
      SPA   A82a;
A829: L     1;
      T     #i;
      SET   ;
      =     #repeatFlag;
      T     #MemFkt;
      L     10;
      T     #SUBSTATE;
      SPA   A828;
A82a: L     10;
      L     LW    22;
      ==I   ;
      SPB   A82b;
      SPA   A82c;
A82b: L     #i;
      L     11;
      <I    ;
      L     #i;
      L     14;
      =     L     18.4;
      >I    ;
      O     L     18.4;
      SPBN  A82d;
      L     #i;
      ITD   ;
      L     L#1;
      >=D   ;
      U     L     18.3;
      =     L     18.3;
      TAK   ;
      L     L#51;
      <=D   ;
      U     L     18.3;
      =     L     18.3;
      TAK   ;
      L     L#1;
      -D    ;
      SPO   I09e;
      SPA   I09f;
I09e: CLR   ;
      =     L     18.3;
I09f: L     L#64;
      *D    ;
      SPO   I0a0;
      SPA   I0a1;
I0a0: CLR   ;
      =     L     18.3;
I0a1: L     L#16;
      +D    ;
      SPO   I0a2;
      SPA   I0a3;
I0a2: CLR   ;
      =     L     18.3;
I0a3: TAR2  ;
      +D    ;
      SPO   I0a4;
      SPA   I0a5;
I0a4: CLR   ;
      =     L     18.3;
I0a5: L     #copyValue;
      TAK   ;
      LAR1  ;
      TAK   ;
      L     DIW [AR1,P#144.0];
      >I    ;
      L     #i;
      ITD   ;
      L     L#1;
      =     L     18.4;
      >=D   ;
      U     L     18.3;
      =     L     18.3;
      TAK   ;
      L     L#51;
      <=D   ;
      U     L     18.3;
      =     L     18.3;
      TAK   ;
      L     L#1;
      -D    ;
      SPO   I0a6;
      SPA   I0a7;
I0a6: CLR   ;
      =     L     18.3;
I0a7: L     L#64;
      *D    ;
      SPO   I0a8;
      SPA   I0a9;
I0a8: CLR   ;
      =     L     18.3;
I0a9: TAR2  ;
      +D    ;
      SPO   I0aa;
      SPA   I0ab;
I0aa: CLR   ;
      =     L     18.3;
I0ab: L     #copyValue;
      TAK   ;
      LAR1  ;
      TAK   ;
      L     DIW [AR1,P#144.0];
      <I    ;
      O     L     18.4;
      =     #tmpBool;
      SPA   A82e;
A82d: L     #i;
      L     -10;
      +I    ;
      SPO   I0ac;
      SPA   I0ad;
I0ac: CLR   ;
      =     L     18.3;
I0ad: ITD   ;
      L     L#1;
      >=D   ;
      U     L     18.3;
      =     L     18.3;
      TAK   ;
      L     L#4;
      <=D   ;
      U     L     18.3;
      =     L     18.3;
      TAK   ;
      L     L#1;
      -D    ;
      SPO   I0ae;
      SPA   I0af;
I0ae: CLR   ;
      =     L     18.3;
I0af: L     L#96;
      *D    ;
      SPO   I0b0;
      SPA   I0b1;
I0b0: CLR   ;
      =     L     18.3;
I0b1: L     L#32;
      +D    ;
      SPO   I0b2;
      SPA   I0b3;
I0b2: CLR   ;
      =     L     18.3;
I0b3: TAR2  ;
      +D    ;
      SPO   I0b4;
      SPA   I0b5;
I0b4: CLR   ;
      =     L     18.3;
I0b5: L     #copyValueLong;
      TAK   ;
      LAR1  ;
      TAK   ;
      L     DID [AR1,P#552.0];
      >D    ;
      L     #i;
      L     -10;
      +I    ;
      =     L     18.4;
      SPO   I0b6;
      SPA   I0b7;
I0b6: CLR   ;
      =     L     18.3;
I0b7: ITD   ;
      L     L#1;
      >=D   ;
      U     L     18.3;
      =     L     18.3;
      TAK   ;
      L     L#4;
      <=D   ;
      U     L     18.3;
      =     L     18.3;
      TAK   ;
      L     L#1;
      -D    ;
      SPO   I0b8;
      SPA   I0b9;
I0b8: CLR   ;
      =     L     18.3;
I0b9: L     L#96;
      *D    ;
      SPO   I0ba;
      SPA   I0bb;
I0ba: CLR   ;
      =     L     18.3;
I0bb: TAR2  ;
      +D    ;
      SPO   I0bc;
      SPA   I0bd;
I0bc: CLR   ;
      =     L     18.3;
I0bd: L     #copyValueLong;
      TAK   ;
      LAR1  ;
      TAK   ;
      L     DID [AR1,P#552.0];
      <D    ;
      O     L     18.4;
      =     #tmpBool;
A82e: CLR   ;
      U     #tmpBool;
      SPBN  A82f;
      CLR   ;
      =     #repeatFlag;
      L     3;
      T     #STATUS;
      L     #i;
      T     #ERROR_LINE;
      L     20;
      T     #INTERNAL_STATE;
      SPA   A828;
A82f: L     #i;
      L     #writeLimit;
      >=I   ;
      SPBN  A831;
      CLR   ;
      =     #repeatFlag;
      SET   ;
      =     #PAR_CHANGE_IN.PARAMODE;
      CLR   ;
      =     #PAR_CHANGE_IN.PARAVALID;
      L     1;
      T     #i;
      L     2;
      T     #STATUS;
      TAK   ;
      T     #MemFkt;
      L     0;
      T     #actWaitCycles;
      L     20;
      T     #SUBSTATE;
      SPA   A832;
A831: SET   ;
      =     #repeatFlag;
      L     #i;
      L     1;
      +I    ;
      SPO   I0be;
      SPA   I0bf;
I0be: CLR   ;
      =     L     18.3;
I0bf: T     #i;
      L     1;
      T     #MemFkt;
A832: SPA   A828;
A82c: L     20;
      L     LW    22;
      ==I   ;
      SPB   A833;
      SPA   A834;
A833: CLR   ;
      U     #PAR_CHANGE_OUT.PARA_ACTIVE;
      SPBN  A835;
      L     30;
      T     #SUBSTATE;
      SPA   A828;
A835: L     #actWaitCycles;
      L     1;
      +I    ;
      SPO   I0c0;
      SPA   I0c1;
I0c0: CLR   ;
      =     L     18.3;
I0c1: T     #actWaitCycles;
      SPA   A828;
A834: L     30;
      L     LW    22;
      ==I   ;
      SPB   A837;
      SPA   A838;
A837: L     0;
      T     #actWaitCycles;
      L     #i;
      L     11;
      <I    ;
      L     #i;
      L     14;
      =     L     18.4;
      >I    ;
      O     L     18.4;
      SPBN  A839;
      L     #copyValue;
      UD    DW#16#FFFF;
      U     L     18.3;
      SAVE  ;
      T     #PAR_CHANGE_IN.PARVAL;
      SPA   A83a;
A839: L     #copyValueLong;
      CLR   ;
      U     L     18.3;
      SAVE  ;
      T     #PAR_CHANGE_IN.PARVAL;
A83a: L     #i;
      ITD   ;
      L     L#1;
      >=D   ;
      U     L     18.3;
      =     L     18.3;
      TAK   ;
      L     L#51;
      <=D   ;
      U     L     18.3;
      =     L     18.3;
      TAK   ;
      L     L#1;
      -D    ;
      SPO   I0c2;
      SPA   I0c3;
I0c2: CLR   ;
      =     L     18.3;
I0c3: L     L#64;
      *D    ;
      SPO   I0c4;
      SPA   I0c5;
I0c4: CLR   ;
      =     L     18.3;
I0c5: L     L#48;
      +D    ;
      SPO   I0c6;
      SPA   I0c7;
I0c6: CLR   ;
      =     L     18.3;
I0c7: TAR2  ;
      +D    ;
      SPO   I0c8;
      SPA   I0c9;
I0c8: CLR   ;
      =     L     18.3;
I0c9: LAR1  ;
      L     DIW [AR1,P#144.0];
      T     #PAR_CHANGE_IN.ADDRESS;
      SET   ;
      =     #PAR_CHANGE_IN.PARAVALID;
      L     40;
      T     #SUBSTATE;
      SPA   A828;
A838: L     40;
      L     LW    22;
      ==I   ;
      SPB   A83b;
      SPA   A83c;
A83b: CLR   ;
      U     #PAR_CHANGE_OUT.PARA_READY;
      SPBN  A83d;
      CLR   ;
      =     #PAR_CHANGE_IN.PARAVALID;
      L     50;
      T     #SUBSTATE;
      L     0;
      T     #actWaitCycles;
      SPA   A828;
A83d: L     #actWaitCycles;
      L     1;
      +I    ;
      SPO   I0ca;
      SPA   I0cb;
I0ca: CLR   ;
      =     L     18.3;
I0cb: T     #actWaitCycles;
      SPA   A828;
A83c: L     50;
      L     LW    22;
      ==I   ;
      SPB   A83f;
      SPA   A840;
A83f: L     0;
      T     #actWaitCycles;
      L     #i;
      L     #writeLimit;
      >=I   ;
      SPBN  A841;
      CLR   ;
      =     #PAR_CHANGE_IN.PARAMODE;
      L     0;
      T     #ERROR_LINE;
      L     60;
      T     #SUBSTATE;
      SPA   A828;
A841: L     #i;
      L     1;
      +I    ;
      SPO   I0cc;
      SPA   I0cd;
I0cc: CLR   ;
      =     L     18.3;
I0cd: T     #i;
      L     1;
      T     #MemFkt;
      L     30;
      T     #SUBSTATE;
      SPA   A828;
A840: L     60;
      L     LW    22;
      ==I   ;
      SPB   A843;
      SPA   A828;
A843: L     #actWaitCycles;
      L     20;
      >=I   ;
      SPBN  A845;
      L     0;
      T     #actWaitCycles;
      T     #SUBSTATE;
      SET   ;
      =     #readOnlyValues;
      L     10;
      T     #INTERNAL_STATE;
      L     1;
      T     #i;
      SPA   A828;
A845: L     #actWaitCycles;
      L     1;
      +I    ;
      SPO   I0ce;
      SPA   I0cf;
I0ce: CLR   ;
      =     L     18.3;
I0cf: T     #actWaitCycles;
A828: SPA   A7d4;
A825: L     40;
      L     LW    20;
      ==I   ;
      SPB   A847;
      SPA   A848;
A847: L     2;
      T     #STATUS;
      L     #SUBSTATE;
      L     0;
      TAK   ;
      ==I   ;
      T     LW    22;
      SPB   A84a;
      SPA   A84b;
A84a: L     #SINGLE_INDEX;
      T     #PAR_CHANGE_IN.ADDRESS;
      CLR   ;
      =     #PAR_CHANGE_IN.READLLIM;
      =     #PAR_CHANGE_IN.READULIM;
      SET   ;
      =     #PAR_CHANGE_IN.PARAREAD;
      L     0;
      T     #actWaitCycles;
      L     #PAR_CHANGE_OUT.PARVAL;
      T     #oldParaReadVal;
      L     10;
      T     #SUBSTATE;
      SPA   A849;
A84b: L     10;
      L     LW    22;
      ==I   ;
      SPB   A84c;
      SPA   A849;
A84c: L     #PAR_CHANGE_OUT.PARVAL;
      L     #oldParaReadVal;
      <>D   ;
      L     #actWaitCycles;
      L     5;
      =     L     18.4;
      >=I   ;
      O     L     18.4;
      SPBN  A84e;
      L     #PAR_CHANGE_OUT.PARVAL;
      T     #SINGLEACCESS;
      U     L     18.3;
      SAVE  ;
      CLR   ;
      =     #PAR_CHANGE_IN.PARAREAD;
      L     0;
      T     #actWaitCycles;
      L     20;
      T     #INTERNAL_STATE;
      L     1;
      T     #STATUS;
      SPA   A849;
A84e: L     #actWaitCycles;
      L     1;
      +I    ;
      SPO   I0d0;
      SPA   I0d1;
I0d0: CLR   ;
      =     L     18.3;
I0d1: T     #actWaitCycles;
A849: SPA   A7d4;
A848: L     50;
      L     LW    20;
      ==I   ;
      SPB   A850;
      SPA   A851;
A850: L     #actWaitCycles;
      L     100;
      >=I   ;
      SPBN  A852;
      L     20;
      T     #INTERNAL_STATE;
      L     -1;
      T     #SUBSTATE;
      L     3;
      T     #STATUS;
      CLR   ;
      =     #PAR_CHANGE_IN.PARAMODE;
      =     #PAR_CHANGE_IN.PARAVALID;
      =     #saveFlag;
      SPA   A853;
A852: L     2;
      T     #STATUS;
A853: L     #SUBSTATE;
      L     0;
      TAK   ;
      ==I   ;
      T     LW    22;
      SPB   A855;
      SPA   A856;
A855: L     2;
      T     #STATUS;
      L     0;
      T     #actWaitCycles;
      L     10;
      T     #SUBSTATE;
      SET   ;
      =     #PAR_CHANGE_IN.PARAMODE;
      SPA   A854;
A856: L     10;
      L     LW    22;
      ==I   ;
      SPB   A857;
      SPA   A858;
A857: CLR   ;
      U     #PAR_CHANGE_OUT.PARA_ACTIVE;
      SPBN  A859;
      L     20;
      T     #SUBSTATE;
      SPA   A854;
A859: L     #actWaitCycles;
      L     1;
      +I    ;
      SPO   I0d2;
      SPA   I0d3;
I0d2: CLR   ;
      =     L     18.3;
I0d3: T     #actWaitCycles;
      SPA   A854;
A858: L     20;
      L     LW    22;
      ==I   ;
      SPB   A85b;
      SPA   A85c;
A85b: L     0;
      T     #actWaitCycles;
      CLR   ;
      U     #saveFlag;
      SPBN  A85d;
      U     L     18.3;
      SAVE  ;
      L     DW#16#3039;
      T     #PAR_CHANGE_IN.PARVAL;
      L     W#16#2222;
      T     #PAR_CHANGE_IN.ADDRESS;
      SPA   A85e;
A85d: L     #SINGLEACCESS;
      CLR   ;
      U     L     18.3;
      SAVE  ;
      T     #PAR_CHANGE_IN.PARVAL;
      L     #SINGLE_INDEX;
      T     #PAR_CHANGE_IN.ADDRESS;
A85e: CLR   ;
      =     #saveFlag;
      SET   ;
      =     #PAR_CHANGE_IN.PARAVALID;
      L     30;
      T     #SUBSTATE;
      SPA   A854;
A85c: L     30;
      L     LW    22;
      ==I   ;
      SPB   A85f;
      SPA   A854;
A85f: CLR   ;
      U     #PAR_CHANGE_OUT.PARA_READY;
      SPBN  A861;
      CLR   ;
      =     #PAR_CHANGE_IN.PARAVALID;
      =     #PAR_CHANGE_IN.PARAMODE;
      L     0;
      T     #SUBSTATE;
      L     20;
      T     #INTERNAL_STATE;
      L     1;
      T     #STATUS;
      L     0;
      T     #actWaitCycles;
      SPA   A854;
A861: L     #actWaitCycles;
      L     1;
      +I    ;
      SPO   I0d4;
      SPA   I0d5;
I0d4: CLR   ;
      =     L     18.3;
I0d5: T     #actWaitCycles;
A854: SPA   A7d4;
A851: L     60;
      L     LW    20;
      ==I   ;
      SPB   A863;
      SPA   A7d4;
A863: L     #actWaitCycles;
      L     100;
      >I    ;
      SPBN  A865;
      L     20;
      T     #INTERNAL_STATE;
      L     -1;
      T     #SUBSTATE;
      L     3;
      T     #STATUS;
      CLR   ;
      =     #PAR_CHANGE_IN.PARAMODE;
      =     #PAR_CHANGE_IN.PARAVALID;
      SPA   A866;
A865: L     2;
      T     #STATUS;
A866: L     #SUBSTATE;
      L     0;
      TAK   ;
      ==I   ;
      T     LW    22;
      SPB   A868;
      SPA   A869;
A868: L     2;
      T     #STATUS;
      L     0;
      T     #actWaitCycles;
      L     10;
      T     #SUBSTATE;
      SET   ;
      =     #PAR_CHANGE_IN.PARAMODE;
      SPA   A867;
A869: L     10;
      L     LW    22;
      ==I   ;
      SPB   A86a;
      SPA   A86b;
A86a: CLR   ;
      U     #PAR_CHANGE_OUT.PARA_ACTIVE;
      SPBN  A86c;
      L     20;
      T     #SUBSTATE;
      SPA   A867;
A86c: L     #actWaitCycles;
      L     1;
      +I    ;
      SPO   I0d6;
      SPA   I0d7;
I0d6: CLR   ;
      =     L     18.3;
I0d7: T     #actWaitCycles;
      SPA   A867;
A86b: L     20;
      L     LW    22;
      ==I   ;
      SPB   A86e;
      SPA   A86f;
A86e: L     0;
      T     #actWaitCycles;
      CLR   ;
      U     L     18.3;
      SAVE  ;
      L     DW#16#3039;
      T     #PAR_CHANGE_IN.PARVAL;
      CLR   ;
      U     #defaultFlag;
      SPBN  A870;
      L     W#16#2233;
      T     #PAR_CHANGE_IN.ADDRESS;
      SPA   A871;
A870: L     W#16#2244;
      T     #PAR_CHANGE_IN.ADDRESS;
A871: SET   ;
      =     #PAR_CHANGE_IN.PARAVALID;
      L     30;
      T     #SUBSTATE;
      SPA   A867;
A86f: L     30;
      L     LW    22;
      ==I   ;
      SPB   A872;
      SPA   A873;
A872: CLR   ;
      U     #PAR_CHANGE_OUT.PARA_READY;
      SPBN  A874;
      CLR   ;
      =     #PAR_CHANGE_IN.PARAVALID;
      =     #PAR_CHANGE_IN.PARAMODE;
      L     40;
      T     #SUBSTATE;
      L     0;
      T     #actWaitCycles;
      SPA   A867;
A874: L     #actWaitCycles;
      L     1;
      +I    ;
      SPO   I0d8;
      SPA   I0d9;
I0d8: CLR   ;
      =     L     18.3;
I0d9: T     #actWaitCycles;
      SPA   A867;
A873: L     40;
      L     LW    22;
      ==I   ;
      SPB   A876;
      SPA   A877;
A876: L     #actWaitCycles;
      L     100;
      >=I   ;
      SPBN  A878;
      L     50;
      T     #SUBSTATE;
      L     0;
      T     #actWaitCycles;
      SPA   A867;
A878: L     #actWaitCycles;
      L     1;
      +I    ;
      SPO   I0da;
      SPA   I0db;
I0da: CLR   ;
      =     L     18.3;
I0db: T     #actWaitCycles;
      SPA   A867;
A877: L     50;
      L     LW    22;
      ==I   ;
      SPB   A87a;
      SPA   A867;
A87a: L     10;
      T     #INTERNAL_STATE;
      L     0;
      T     #SUBSTATE;
      L     1;
      T     #i;
      SET   ;
      =     #readOnlyValues;
A867: CLR   ;
A7d4: CLR   ;
      U     #READ_ALL;
      =     #oldREADALL;
      U     #WRITE_SEL;
      =     #oldWRITESEL;
      U     #WRITE_ALL;
      =     #oldWRITEALL;
      U     #SINGLE_READ;
      =     #oldSINGLEREAD;
      U     #SINGLE_WRITE;
      =     #oldSINGLEWRITE;
      U     #SAVE;
      =     #oldSAVE;
      U     #DEFAULT;
      =     #oldDEFAULT;
      U     #LOADBACK;
      =     #oldLOADBACK;
      U     #PAR_CHANGE_OUT.PARA_READY;
      =     #oldPARAREADY;
      L     #MemFkt;
      L     1;
      TAK   ;
      ==I   ;
      T     LW    20;
      SPB   A87d;
      SPA   A87e;
A87d: L     #i;
      L     1;
      TAK   ;
      ==I   ;
      T     LW    22;
      SPB   A880;
      SPA   A881;
A880: L     9999;
      T     #copyValue;
      L     1;
      T     #k;
A882: L     #k;
      L     14;
      <=I   ;
      SPBN  A87f;
      L     #k;
      ITD   ;
      L     L#1;
      >=D   ;
      U     L     18.3;
      =     L     18.3;
      TAK   ;
      L     L#15;
      <=D   ;
      U     L     18.3;
      =     L     18.3;
      TAK   ;
      L     L#1;
      -D    ;
      SPO   I0dc;
      SPA   I0dd;
I0dc: CLR   ;
      =     L     18.3;
I0dd: L     L#16;
      *D    ;
      SPO   I0de;
      SPA   I0df;
I0de: CLR   ;
      =     L     18.3;
I0df: TAR2  ;
      +D    ;
      SPO   I0e0;
      SPA   I0e1;
I0e0: CLR   ;
      =     L     18.3;
I0e1: LAR1  ;
      L     DIW [AR1,P#624.0];
      L     #PVSEL;
      ==I   ;
      SPBN  A884;
      L     #k;
      T     #copyValue;
A884: L     #k;
      L     1;
      +I    ;
      SPO   I0e2;
      SPA   I0e3;
I0e2: CLR   ;
      =     L     18.3;
I0e3: T     #k;
      SPA   A882;
      SPA   A87f;
A881: L     2;
      L     LW    22;
      ==I   ;
      SPB   A885;
      SPA   A886;
A885: L     #PTYPE;
      T     #copyValue;
      SPA   A87f;
A886: L     3;
      L     LW    22;
      ==I   ;
      SPB   A887;
      SPA   A888;
A887: L     #CO;
      T     #copyValue;
      SPA   A87f;
A888: L     4;
      L     LW    22;
      ==I   ;
      SPB   A889;
      SPA   A88a;
A889: L     #DSP_VALVE;
      T     #copyValue;
      SPA   A87f;
A88a: L     5;
      L     LW    22;
      ==I   ;
      SPB   A88b;
      SPA   A88c;
A88b: L     #PSENSOR;
      T     #copyValue;
      SPA   A87f;
A88c: L     6;
      L     LW    22;
      ==I   ;
      SPB   A88d;
      SPA   A88e;
A88d: L     #PNOMINAL;
      T     #copyValue;
      SPA   A87f;
A88e: L     7;
      L     LW    22;
      ==I   ;
      SPB   A88f;
      SPA   A890;
A88f: L     #PCORR;
      T     #copyValue;
      SPA   A87f;
A890: L     8;
      L     LW    22;
      ==I   ;
      SPB   A891;
      SPA   A892;
A891: L     #PLRPM;
      T     #copyValue;
      SPA   A87f;
A892: L     9;
      L     LW    22;
      ==I   ;
      SPB   A893;
      SPA   A894;
A893: L     #PLPL;
      T     #copyValue;
      SPA   A87f;
A894: L     10;
      L     LW    22;
      ==I   ;
      SPB   A895;
      SPA   A896;
A895: L     #QCORR;
      T     #copyValue;
      SPA   A87f;
A896: L     11;
      L     LW    22;
      ==I   ;
      SPB   A897;
      SPA   A898;
A897: L     #AQUP;
      T     #copyValueLong;
      SPA   A87f;
A898: L     12;
      L     LW    22;
      ==I   ;
      SPB   A899;
      SPA   A89a;
A899: L     #AQDOWN;
      T     #copyValueLong;
      SPA   A87f;
A89a: L     13;
      L     LW    22;
      ==I   ;
      SPB   A89b;
      SPA   A89c;
A89b: L     #APUP;
      T     #copyValueLong;
      SPA   A87f;
A89c: L     14;
      L     LW    22;
      ==I   ;
      SPB   A89d;
      SPA   A89e;
A89d: L     #APDOWN;
      T     #copyValueLong;
      SPA   A87f;
A89e: L     15;
      L     LW    22;
      ==I   ;
      SPB   A89f;
      SPA   A8a0;
A89f: L     #MINXQ;
      T     #copyValue;
      SPA   A87f;
A8a0: L     16;
      L     LW    22;
      ==I   ;
      SPB   A8a1;
      SPA   A8a2;
A8a1: L     #MAXXQ;
      T     #copyValue;
      SPA   A87f;
A8a2: L     17;
      L     LW    22;
      ==I   ;
      SPB   A8a3;
      SPA   A8a4;
A8a3: L     #AINXQ;
      T     #copyValue;
      SPA   A87f;
A8a4: L     18;
      L     LW    22;
      ==I   ;
      SPB   A8a5;
      SPA   A8a6;
A8a5: L     #AINXP;
      T     #copyValue;
      SPA   A87f;
A8a6: L     19;
      L     LW    22;
      ==I   ;
      SPB   A8a7;
      SPA   A8a8;
A8a7: L     #CQFF;
      T     #copyValue;
      SPA   A87f;
A8a8: L     20;
      L     LW    22;
      ==I   ;
      SPB   A8a9;
      SPA   A8aa;
A8a9: L     #CQP;
      T     #copyValue;
      SPA   A87f;
A8aa: L     21;
      L     LW    22;
      ==I   ;
      SPB   A8ab;
      SPA   A8ac;
A8ab: L     #CQI;
      T     #copyValue;
      SPA   A87f;
A8ac: L     22;
      L     LW    22;
      ==I   ;
      SPB   A8ad;
      SPA   A8ae;
A8ad: L     #CQILIM;
      T     #copyValue;
      SPA   A87f;
A8ae: L     23;
      L     LW    22;
      ==I   ;
      SPB   A8af;
      SPA   A8b0;
A8af: L     #CQIC;
      T     #copyValue;
      SPA   A87f;
A8b0: L     24;
      L     LW    22;
      ==I   ;
      SPB   A8b1;
      SPA   A8b2;
A8b1: L     #CQD;
      T     #copyValue;
      SPA   A87f;
A8b2: L     25;
      L     LW    22;
      ==I   ;
      SPB   A8b3;
      SPA   A8b4;
A8b3: L     #CQT1;
      T     #copyValue;
      SPA   A87f;
A8b4: L     26;
      L     LW    22;
      ==I   ;
      SPB   A8b5;
      SPA   A8b6;
A8b5: L     #CPFF;
      T     #copyValue;
      SPA   A87f;
A8b6: L     27;
      L     LW    22;
      ==I   ;
      SPB   A8b7;
      SPA   A8b8;
A8b7: L     #CPP;
      T     #copyValue;
      SPA   A87f;
A8b8: L     28;
      L     LW    22;
      ==I   ;
      SPB   A8b9;
      SPA   A8ba;
A8b9: L     #CPI;
      T     #copyValue;
      SPA   A87f;
A8ba: L     29;
      L     LW    22;
      ==I   ;
      SPB   A8bb;
      SPA   A8bc;
A8bb: L     #CPILIM;
      T     #copyValue;
      SPA   A87f;
A8bc: L     30;
      L     LW    22;
      ==I   ;
      SPB   A8bd;
      SPA   A8be;
A8bd: L     #CPIC;
      T     #copyValue;
      SPA   A87f;
A8be: L     31;
      L     LW    22;
      ==I   ;
      SPB   A8bf;
      SPA   A8c0;
A8bf: L     #CPD;
      T     #copyValue;
      SPA   A87f;
A8c0: L     32;
      L     LW    22;
      ==I   ;
      SPB   A8c1;
      SPA   A8c2;
A8c1: L     #CPT1;
      T     #copyValue;
      SPA   A87f;
A8c2: L     33;
      L     LW    22;
      ==I   ;
      SPB   A8c3;
      SPA   A8c4;
A8c3: L     #CQMINVA;
      T     #copyValue;
      SPA   A87f;
A8c4: L     34;
      L     LW    22;
      ==I   ;
      SPB   A8c5;
      SPA   A8c6;
A8c5: L     #CQMINVB;
      T     #copyValue;
      SPA   A87f;
A8c6: L     35;
      L     LW    22;
      ==I   ;
      SPB   A8c7;
      SPA   A8c8;
A8c7: L     #CQMAXVA;
      T     #copyValue;
      SPA   A87f;
A8c8: L     36;
      L     LW    22;
      ==I   ;
      SPB   A8c9;
      SPA   A8ca;
A8c9: L     #CQMAXVB;
      T     #copyValue;
      SPA   A87f;
A8ca: L     37;
      L     LW    22;
      ==I   ;
      SPB   A8cb;
      SPA   A8cc;
A8cb: L     #TRIGGERQ;
      T     #copyValue;
      SPA   A87f;
A8cc: L     38;
      L     LW    22;
      ==I   ;
      SPB   A8cd;
      SPA   A8ce;
A8cd: L     #OFFSETQ;
      T     #copyValue;
      SPA   A87f;
A8ce: L     39;
      L     LW    22;
      ==I   ;
      SPB   A8cf;
      SPA   A8d0;
A8cf: L     #CPMINV;
      T     #copyValue;
      SPA   A87f;
A8d0: L     40;
      L     LW    22;
      ==I   ;
      SPB   A8d1;
      SPA   A8d2;
A8d1: L     #CPMAXV;
      T     #copyValue;
      SPA   A87f;
A8d2: L     41;
      L     LW    22;
      ==I   ;
      SPB   A8d3;
      SPA   A8d4;
A8d3: L     #TRIGGERP;
      T     #copyValue;
      SPA   A87f;
A8d4: L     42;
      L     LW    22;
      ==I   ;
      SPB   A8d5;
      SPA   A8d6;
A8d5: L     #DFREQQ;
      T     #copyValue;
      SPA   A87f;
A8d6: L     43;
      L     LW    22;
      ==I   ;
      SPB   A8d7;
      SPA   A8d8;
A8d7: L     #DAMPLQ;
      T     #copyValue;
      SPA   A87f;
A8d8: L     44;
      L     LW    22;
      ==I   ;
      SPB   A8d9;
      SPA   A8da;
A8d9: L     #PWMQ;
      T     #copyValue;
      SPA   A87f;
A8da: L     45;
      L     LW    22;
      ==I   ;
      SPB   A8db;
      SPA   A8dc;
A8db: L     #PPWMQ;
      T     #copyValue;
      SPA   A87f;
A8dc: L     46;
      L     LW    22;
      ==I   ;
      SPB   A8dd;
      SPA   A8de;
A8dd: L     #IPWMQ;
      T     #copyValue;
      SPA   A87f;
A8de: L     47;
      L     LW    22;
      ==I   ;
      SPB   A8df;
      SPA   A8e0;
A8df: L     #DFREQP;
      T     #copyValue;
      SPA   A87f;
A8e0: L     48;
      L     LW    22;
      ==I   ;
      SPB   A8e1;
      SPA   A8e2;
A8e1: L     #DAMPLP;
      T     #copyValue;
      SPA   A87f;
A8e2: L     49;
      L     LW    22;
      ==I   ;
      SPB   A8e3;
      SPA   A8e4;
A8e3: L     #PWMP;
      T     #copyValue;
      SPA   A87f;
A8e4: L     50;
      L     LW    22;
      ==I   ;
      SPB   A8e5;
      SPA   A8e6;
A8e5: L     #PPWMP;
      T     #copyValue;
      SPA   A87f;
A8e6: L     51;
      L     LW    22;
      ==I   ;
      SPB   A8e7;
      SPA   A87f;
A8e7: L     #IPWMP;
      T     #copyValue;
A87f: SPA   A87c;
A87e: L     2;
      L     LW    20;
      ==I   ;
      SPB   A8e9;
      SPA   A87c;
A8e9: L     #i;
      L     1;
      TAK   ;
      ==I   ;
      T     LW    22;
      SPB   A8ec;
      SPA   A8ed;
A8ec: L     #copyValue;
      ITD   ;
      L     L#1;
      >=D   ;
      U     L     18.3;
      =     L     18.3;
      TAK   ;
      L     L#15;
      <=D   ;
      U     L     18.3;
      =     L     18.3;
      TAK   ;
      L     L#1;
      -D    ;
      SPO   I0e4;
      SPA   I0e5;
I0e4: CLR   ;
      =     L     18.3;
I0e5: L     L#16;
      *D    ;
      SPO   I0e6;
      SPA   I0e7;
I0e6: CLR   ;
      =     L     18.3;
I0e7: TAR2  ;
      +D    ;
      SPO   I0e8;
      SPA   I0e9;
I0e8: CLR   ;
      =     L     18.3;
I0e9: LAR1  ;
      L     DIW [AR1,P#624.0];
      T     #PVSEL;
      SPA   A8eb;
A8ed: L     2;
      L     LW    22;
      ==I   ;
      SPB   A8ee;
      SPA   A8ef;
A8ee: L     #copyValue;
      T     #PTYPE;
      SPA   A8eb;
A8ef: L     3;
      L     LW    22;
      ==I   ;
      SPB   A8f0;
      SPA   A8f1;
A8f0: L     #copyValue;
      T     #CO;
      SPA   A8eb;
A8f1: L     4;
      L     LW    22;
      ==I   ;
      SPB   A8f2;
      SPA   A8f3;
A8f2: L     #copyValue;
      T     #DSP_VALVE;
      SPA   A8eb;
A8f3: L     5;
      L     LW    22;
      ==I   ;
      SPB   A8f4;
      SPA   A8f5;
A8f4: L     #copyValue;
      T     #PSENSOR;
      SPA   A8eb;
A8f5: L     6;
      L     LW    22;
      ==I   ;
      SPB   A8f6;
      SPA   A8f7;
A8f6: L     #copyValue;
      T     #PNOMINAL;
      SPA   A8eb;
A8f7: L     7;
      L     LW    22;
      ==I   ;
      SPB   A8f8;
      SPA   A8f9;
A8f8: L     #copyValue;
      T     #PCORR;
      SPA   A8eb;
A8f9: L     8;
      L     LW    22;
      ==I   ;
      SPB   A8fa;
      SPA   A8fb;
A8fa: L     #copyValue;
      T     #PLRPM;
      SPA   A8eb;
A8fb: L     9;
      L     LW    22;
      ==I   ;
      SPB   A8fc;
      SPA   A8fd;
A8fc: L     #copyValue;
      T     #PLPL;
      SPA   A8eb;
A8fd: L     10;
      L     LW    22;
      ==I   ;
      SPB   A8fe;
      SPA   A8ff;
A8fe: L     #copyValue;
      T     #QCORR;
      SPA   A8eb;
A8ff: L     11;
      L     LW    22;
      ==I   ;
      SPB   A900;
      SPA   A901;
A900: L     #copyValueLong;
      T     #AQUP;
      SPA   A8eb;
A901: L     12;
      L     LW    22;
      ==I   ;
      SPB   A902;
      SPA   A903;
A902: L     #copyValueLong;
      T     #AQDOWN;
      SPA   A8eb;
A903: L     13;
      L     LW    22;
      ==I   ;
      SPB   A904;
      SPA   A905;
A904: L     #copyValueLong;
      T     #APUP;
      SPA   A8eb;
A905: L     14;
      L     LW    22;
      ==I   ;
      SPB   A906;
      SPA   A907;
A906: L     #copyValueLong;
      T     #APDOWN;
      SPA   A8eb;
A907: L     15;
      L     LW    22;
      ==I   ;
      SPB   A908;
      SPA   A909;
A908: L     #copyValue;
      T     #MINXQ;
      SPA   A8eb;
A909: L     16;
      L     LW    22;
      ==I   ;
      SPB   A90a;
      SPA   A90b;
A90a: L     #copyValue;
      T     #MAXXQ;
      SPA   A8eb;
A90b: L     17;
      L     LW    22;
      ==I   ;
      SPB   A90c;
      SPA   A90d;
A90c: L     #copyValue;
      T     #AINXQ;
      SPA   A8eb;
A90d: L     18;
      L     LW    22;
      ==I   ;
      SPB   A90e;
      SPA   A90f;
A90e: L     #copyValue;
      T     #AINXP;
      SPA   A8eb;
A90f: L     19;
      L     LW    22;
      ==I   ;
      SPB   A910;
      SPA   A911;
A910: L     #copyValue;
      T     #CQFF;
      SPA   A8eb;
A911: L     20;
      L     LW    22;
      ==I   ;
      SPB   A912;
      SPA   A913;
A912: L     #copyValue;
      T     #CQP;
      SPA   A8eb;
A913: L     21;
      L     LW    22;
      ==I   ;
      SPB   A914;
      SPA   A915;
A914: L     #copyValue;
      T     #CQI;
      SPA   A8eb;
A915: L     22;
      L     LW    22;
      ==I   ;
      SPB   A916;
      SPA   A917;
A916: L     #copyValue;
      T     #CQILIM;
      SPA   A8eb;
A917: L     23;
      L     LW    22;
      ==I   ;
      SPB   A918;
      SPA   A919;
A918: L     #copyValue;
      T     #CQIC;
      SPA   A8eb;
A919: L     24;
      L     LW    22;
      ==I   ;
      SPB   A91a;
      SPA   A91b;
A91a: L     #copyValue;
      T     #CQD;
      SPA   A8eb;
A91b: L     25;
      L     LW    22;
      ==I   ;
      SPB   A91c;
      SPA   A91d;
A91c: L     #copyValue;
      T     #CQT1;
      SPA   A8eb;
A91d: L     26;
      L     LW    22;
      ==I   ;
      SPB   A91e;
      SPA   A91f;
A91e: L     #copyValue;
      T     #CPFF;
      SPA   A8eb;
A91f: L     27;
      L     LW    22;
      ==I   ;
      SPB   A920;
      SPA   A921;
A920: L     #copyValue;
      T     #CPP;
      SPA   A8eb;
A921: L     28;
      L     LW    22;
      ==I   ;
      SPB   A922;
      SPA   A923;
A922: L     #copyValue;
      T     #CPI;
      SPA   A8eb;
A923: L     29;
      L     LW    22;
      ==I   ;
      SPB   A924;
      SPA   A925;
A924: L     #copyValue;
      T     #CPILIM;
      SPA   A8eb;
A925: L     30;
      L     LW    22;
      ==I   ;
      SPB   A926;
      SPA   A927;
A926: L     #copyValue;
      T     #CPIC;
      SPA   A8eb;
A927: L     31;
      L     LW    22;
      ==I   ;
      SPB   A928;
      SPA   A929;
A928: L     #copyValue;
      T     #CPD;
      SPA   A8eb;
A929: L     32;
      L     LW    22;
      ==I   ;
      SPB   A92a;
      SPA   A92b;
A92a: L     #copyValue;
      T     #CPT1;
      SPA   A8eb;
A92b: L     33;
      L     LW    22;
      ==I   ;
      SPB   A92c;
      SPA   A92d;
A92c: L     #copyValue;
      T     #CQMINVA;
      SPA   A8eb;
A92d: L     34;
      L     LW    22;
      ==I   ;
      SPB   A92e;
      SPA   A92f;
A92e: L     #copyValue;
      T     #CQMINVB;
      SPA   A8eb;
A92f: L     35;
      L     LW    22;
      ==I   ;
      SPB   A930;
      SPA   A931;
A930: L     #copyValue;
      T     #CQMAXVA;
      SPA   A8eb;
A931: L     36;
      L     LW    22;
      ==I   ;
      SPB   A932;
      SPA   A933;
A932: L     #copyValue;
      T     #CQMAXVB;
      SPA   A8eb;
A933: L     37;
      L     LW    22;
      ==I   ;
      SPB   A934;
      SPA   A935;
A934: L     #copyValue;
      T     #TRIGGERQ;
      SPA   A8eb;
A935: L     38;
      L     LW    22;
      ==I   ;
      SPB   A936;
      SPA   A937;
A936: L     #copyValue;
      T     #OFFSETQ;
      SPA   A8eb;
A937: L     39;
      L     LW    22;
      ==I   ;
      SPB   A938;
      SPA   A939;
A938: L     #copyValue;
      T     #CPMINV;
      SPA   A8eb;
A939: L     40;
      L     LW    22;
      ==I   ;
      SPB   A93a;
      SPA   A93b;
A93a: L     #copyValue;
      T     #CPMAXV;
      SPA   A8eb;
A93b: L     41;
      L     LW    22;
      ==I   ;
      SPB   A93c;
      SPA   A93d;
A93c: L     #copyValue;
      T     #TRIGGERP;
      SPA   A8eb;
A93d: L     42;
      L     LW    22;
      ==I   ;
      SPB   A93e;
      SPA   A93f;
A93e: L     #copyValue;
      T     #DFREQQ;
      SPA   A8eb;
A93f: L     43;
      L     LW    22;
      ==I   ;
      SPB   A940;
      SPA   A941;
A940: L     #copyValue;
      T     #DAMPLQ;
      SPA   A8eb;
A941: L     44;
      L     LW    22;
      ==I   ;
      SPB   A942;
      SPA   A943;
A942: L     #copyValue;
      T     #PWMQ;
      SPA   A8eb;
A943: L     45;
      L     LW    22;
      ==I   ;
      SPB   A944;
      SPA   A945;
A944: L     #copyValue;
      T     #PPWMQ;
      SPA   A8eb;
A945: L     46;
      L     LW    22;
      ==I   ;
      SPB   A946;
      SPA   A947;
A946: L     #copyValue;
      T     #IPWMQ;
      SPA   A8eb;
A947: L     47;
      L     LW    22;
      ==I   ;
      SPB   A948;
      SPA   A949;
A948: L     #copyValue;
      T     #DFREQP;
      SPA   A8eb;
A949: L     48;
      L     LW    22;
      ==I   ;
      SPB   A94a;
      SPA   A94b;
A94a: L     #copyValue;
      T     #DAMPLP;
      SPA   A8eb;
A94b: L     49;
      L     LW    22;
      ==I   ;
      SPB   A94c;
      SPA   A94d;
A94c: L     #copyValue;
      T     #PWMP;
      SPA   A8eb;
A94d: L     50;
      L     LW    22;
      ==I   ;
      SPB   A94e;
      SPA   A94f;
A94e: L     #copyValue;
      T     #PPWMP;
      SPA   A8eb;
A94f: L     51;
      L     LW    22;
      ==I   ;
      SPB   A950;
      SPA   A8eb;
A950: L     #copyValue;
      T     #IPWMP;
A8eb: CLR   ;
A87c: L     0;
      T     #MemFkt;
      CLR   ;
      U     #repeatFlag;
      NOT   ;
      SPBN  A7d0;
      U     L     18.3;
      SAVE  ;
      BE    ;
END_FUNCTION_BLOCK

